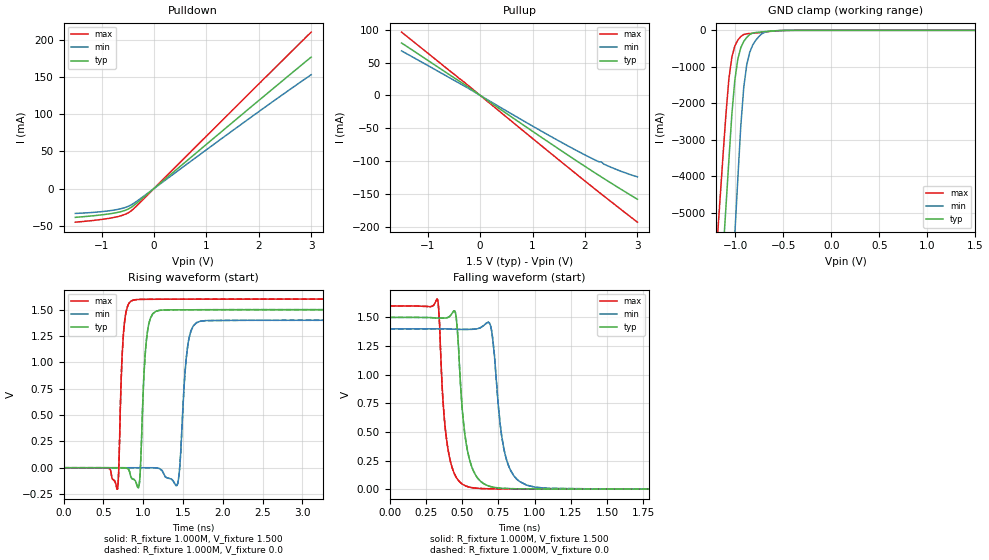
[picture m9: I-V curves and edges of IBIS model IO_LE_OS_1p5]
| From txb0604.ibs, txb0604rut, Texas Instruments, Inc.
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|   Model IO_LE_OS_1p5
[Model] IO_LE_OS_1p5
Model_type 3-state
Polarity   Non-Inverting
Enable   Active-High
Vmeas =  0.750V
Cref =  15.000pF
Rref =  1.000M
Vref =  0.0V
C_comp   3.930pF   3.640pF   4.130pF
[Temperature Range]   27.000   0.125k   -40.000
[Voltage Range]   1.500V   1.400V   1.600V
[Pullup Reference]   1.500V   1.400V   1.600V
[Pulldown Reference]   0.0V   0.0V   0.0V
[POWER Clamp Reference]   1.500V   1.400V   1.600V
[GND Clamp Reference]   0.0V   0.0V   0.0V
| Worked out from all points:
|   slope of the pulldown table from 0 to 0.225 V, typ, clamps not added: 16.8 ohm
|   slope of the pullup table from 0 to 0.225 V, typ, clamps not added: 18.1 ohm
|   GND clamp passes 1 mA (typ) near -0.43 V on its own axis
|   rising waveform, R_fixture 1.000M, V_fixture 1.500: 20-80 % time 58.9ps typ, 72.8ps min, 47.8ps max; typ from 0 V to 1.5 V
|   rising waveform, R_fixture 1.000M, V_fixture 0.0: 20-80 % time 58.9ps typ, 72.8ps min, 47.8ps max; typ from 0 V to 1.5 V
|   falling waveform, R_fixture 1.000M, V_fixture 1.500: 20-80 % time 66.3ps typ, 75.7ps min, 57.4ps max; typ from 1.5 V to 0 V
|   falling waveform, R_fixture 1.000M, V_fixture 0.0: 20-80 % time 66.3ps typ, 75.7ps min, 57.4ps max; typ from 1.5 V to 0 V
[Pulldown]
|Voltage   I(typ)   I(min)   I(max)
-1.5V     -38.78mA   -33.47mA   -45.28mA
-764mV    -33.07mA   -28.96mA   -38.92mA
-580mV    -30.08mA   -26.17mA   -35.49mA
-442mV    -25.69mA   -22.29mA   -30.48mA
2.042V    121.1mA    105.8mA    143.8mA
3V        177.1mA    153.4mA    210.8mA
[Pullup]
|Voltage   I(typ)   I(min)   I(max)
-1.5V     79.89mA    67.84mA    96.48mA
-312mV    17.19mA    14.74mA    20.59mA
930mV     -50.97mA   -43.6mA    -61.14mA
1.804V    -97.93mA   -82.58mA   -118mA
2.264V    -121.9mA   -101.2mA   -147.4mA
2.31V     -124.2mA   -101.4mA   -150.3mA
2.402V    -128.9mA   -106.3mA   -156.1mA
3V        -158.3mA   -124.2mA   -193.3mA
[GND_clamp]
|Voltage   I(typ)   I(min)   I(max)
-1.5V     -21.77A    -29.65A    -17.82A
-1.19V    -8.766A    -14.61A    -5.864A
-1.159V   -7.466A    -13.1A     -4.668A
-1.128V   -6.165A    -11.6A     -3.473A
-1.097V   -4.864A    -10.09A    -2.32A
-1.066V   -3.563A    -8.59A     -1.334A
-1.004V   -1.365A    -5.582A    -426.6mA
-911mV    -303.9mA   -1.56A     -113.8mA
-880mV    -195.6mA   -944.5mA   -95.38mA
-818mV    -75mA      -403.2mA   -78.97mA
-663mV    -28.8mA    -34.23mA   -37.49mA
1.5V      0A         0A         0A
[Ramp]
| variable   typ   min   max
dV/dt_r   0.900/59.019p   0.840/72.708p   0.960/48.186p
dV/dt_f   0.900/66.951p   0.840/76.617p   0.960/57.158p
R_load = 1.000M
[Rising Waveform]
R_fixture= 1.000M
V_fixture= 1.500
V_fixture_min= 1.400
V_fixture_max= 1.600
|time   V(typ)   V(min)   V(max)
0s        25.1uV     28.78uV    22.56uV
678ps     -77.34uV   11.24uV    -202mV
757ps     -397.9uV   -1.108uV   1.312V
885ps     -111.1mV   -42.2uV    1.592V
1.06ns    1.321V     -37.42uV   1.598V
1.204ns   1.493V     -7.239mV   1.598V
1.435ns   1.498V     -146.2mV   1.599V
1.559ns   1.498V     1.152V     1.599V
1.719ns   1.499V     1.39V      1.599V
10ns      1.5V       1.4V       1.6V
[Rising Waveform]
R_fixture= 1.000M
V_fixture= 0.0
V_fixture_min= 0.0
V_fixture_max= 0.0
|time   V(typ)   V(min)   V(max)
0s        -28.12nV   2.123uV    -68.74nV
678ps     -102.5uV   -15.42uV   -202.1mV
757ps     -423.3uV   -27.76uV   1.312V
885ps     -111.2mV   -68.87uV   1.592V
1.06ns    1.321V     -64.22uV   1.598V
1.204ns   1.493V     -7.267mV   1.598V
1.435ns   1.498V     -146.3mV   1.599V
1.559ns   1.498V     1.152V     1.599V
1.719ns   1.499V     1.39V      1.599V
10ns      1.5V       1.4V       1.6V
[Falling Waveform]
R_fixture= 1.000M
V_fixture= 1.500
V_fixture_min= 1.400
V_fixture_max= 1.600
|time   V(typ)   V(min)   V(max)
0s        1.5V       1.4V       1.6V
331ps     1.494V     1.4V       1.651V
381ps     1.494V     1.4V       552.8mV
448ps     1.556V     1.397V     130.1mV
516ps     499.4mV    1.395V     33.04mV
576ps     162.8mV    1.397V     11.57mV
695ps     23.02mV    1.429V     3.374mV
805ps     5.707mV    260.2mV    2.259mV
1.005ns   2.167mV    16.69mV    1.444mV
10ns      32.29uV    45.53uV    24.39uV
[Falling Waveform]
R_fixture= 1.000M
V_fixture= 0.0
V_fixture_min= 0.0
V_fixture_max= 0.0
|time   V(typ)   V(min)   V(max)
0s        1.5V       1.4V       1.6V
331ps     1.494V     1.4V       1.651V
381ps     1.494V     1.4V       552.8mV
448ps     1.556V     1.397V     130mV
516ps     499.3mV    1.395V     33.01mV
576ps     162.8mV    1.397V     11.54mV
695ps     23mV       1.429V     3.352mV
805ps     5.681mV    260.1mV    2.236mV
1.005ns   2.142mV    16.67mV    1.422mV
10ns      7.157uV    18.88uV    1.764uV
